DATA_BLOCK DB 1
TITLE =Analog value display
VERSION : 0.1


  STRUCT
   CH_0 : INT ; //Channel 0
   CH_1 : INT ; //Channel 1
   CH_2 : INT ; //Channel 2
   CH_3 : INT ; //Channel 3
   CH_4 : INT ; //Channel 4
   CH_5 : INT ; //Channel 5
   CH_6 : INT ; //Channel 6
   CH_7 : INT ; //Channel 7
  END_STRUCT ;
BEGIN
   CH_0 := 0;
   CH_1 := 0;
   CH_2 := 0;
   CH_3 := 0;
   CH_4 := 0;
   CH_5 := 0;
   CH_6 := 0;
   CH_7 := 0;
END_DATA_BLOCK

DATA_BLOCK DB 2
TITLE =Process values
VERSION : 0.1

  STRUCT
   SE_1 : REAL ;    //Voltage Transducer
   SE_2 : REAL ;    //PT100 (4)
   SE_3 : REAL ;    //PT100 (3)
   SE_4 : REAL ;    //PT100 (2)
  END_STRUCT ;
BEGIN
   SE_1 := 0.000000e+000;
   SE_2 := 0.000000e+000;
   SE_3 := 0.000000e+000;
   SE_4 := 0.000000e+000;
END_DATA_BLOCK

FUNCTION FC 1 : VOID
TITLE =Convert analog value display to process values
VERSION : 0.1


VAR_INPUT
  RawValue : INT ;
  Factor : REAL ;
  Offset : REAL ;
  OverFlow : INT ;
  OverRange : INT ;
  UnderRange : INT ;
  UnderFlow : INT ;
END_VAR
VAR_OUTPUT
  MeasuredValue : REAL ;
  Status : WORD ;
END_VAR
VAR_TEMP
  TInt : INT ;
  TDoubleInt : DINT ;
  TFactor : REAL ;
  TOffset : REAL ;
  TFactor1 : DINT ;
  TFactor2 : REAL ;
END_VAR
BEGIN
NETWORK
TITLE =Conversion

      L     #RawValue;
      ITD   ;
      DTR   ;
      L     #Factor;
      *R    ;
      L     #Offset;
      +R    ;
      T     #MeasuredValue;

NETWORK
TITLE =Analog value display monitoring

      L     W#16#0;
      T     #Status;


      L     #RawValue;
      L     #OverFlow;
      >=I   ;
      SPB   m_of;

      L     #RawValue;
      L     #OverRange;
      >=I   ;
      SPB   m_or;

      L     #RawValue;
      L     #UnderFlow;
      <=I   ;
      SPB   m_uf;

      L     #RawValue;
      L     #UnderRange;
      <=I   ;
      SPB   m_ur;

      SPA   end;

m_of: L     W#16#800;
      T     #Status;
      SPA   end;

m_or: L     W#16#400;
      T     #Status;
      SPA   end;

m_uf: L     W#16#200;
      T     #Status;
      SPA   end;

m_ur: L     W#16#100;
      T     #Status;
      SPA   end;

end:  NOP   0;
END_FUNCTION

ORGANIZATION_BLOCK OB 1
TITLE = "Main Program Sweep (Cycle)"
VERSION : 0.1


VAR_TEMP
  OB1_EV_CLASS : BYTE ; //Bits 0-3 = 1 (Coming event), Bits 4-7 = 1 (Event class 1)
  OB1_SCAN_1 : BYTE ;   //1 (Cold restart scan 1 of OB 1), 3 (Scan 2-n of OB 1)
  OB1_PRIORITY : BYTE ; //Priority of OB Execution
  OB1_OB_NUMBR : BYTE ; //1 (Organization block 1, OB1)
  OB1_RESERVED_1 : BYTE ;   //Reserved for system
  OB1_RESERVED_2 : BYTE ;   //Reserved for system
  OB1_PREV_CYCLE : INT ;    //Cycle time of previous OB1 scan (millisec-onds)
  OB1_MIN_CYCLE : INT ; //Minimum cycle time of OB1 (milliseconds)
  OB1_MAX_CYCLE : INT ; //Maximum cycle time of OB1 (milliseconds)
  OB1_DATE_TIME : DATE_AND_TIME ;   //Date and time OB1 started
END_VAR
BEGIN
NETWORK
TITLE =Transfer of channel values into data block DB1

// Channel 0 -> Data block
      L     PIW  352;
      T     DB1.DBW    0;

// Channel 1 -> Data block
      L     PIW  354;
      T     DB1.DBW    2;

// Channel 2 -> Data block
      L     PIW  356;
      T     DB1.DBW    4;

// Channel 3 -> Data block
      L     PIW  358;
      T     DB1.DBW    6;

// Channel 4 -> Data block
      L     PIW  360;
      T     DB1.DBW    8;

// Channel 5 -> Data block
      L     PIW  362;
      T     DB1.DBW   10;

// Channel 6 -> Data block
      L     PIW  364;
      T     DB1.DBW   12;

// Channel 7 -> Data block
      L     PIW  366;
      T     DB1.DBW   14;



NETWORK
TITLE =Converting analog value display -> Measurement value

// Channel 1 : Voltage transducer 1 to 5V

      CALL FC     1 (
           RawValue                 := DB1.DBW    0,
           Factor                   := 1.447000e-004,
           Offset                   := 1.000000e+000,
           OverFlow                 := 32512,
           OverRange                := 27649,
           UnderRange               := -1,
           UnderFlow                := -4865,
           MeasuredValue            := DB2.DBD    0,
           Status                   := MW    10);

// Channel 2 : PT100

      CALL FC     1 (
           RawValue                 := DB1.DBW    4,
           Factor                   := 1.000000e-001,
           Offset                   := 0.000000e+000,
           OverFlow                 := 10001,
           OverRange                := 8501,
           UnderRange               := -2001,
           UnderFlow                := -2431,
           MeasuredValue            := DB2.DBD    4,
           Status                   := MW    20);

// Channel 3 : PT100

      CALL FC     1 (
           RawValue                 := DB1.DBW    8,
           Factor                   := 1.000000e-001,
           Offset                   := 0.000000e+000,
           OverFlow                 := 10001,
           OverRange                := 8501,
           UnderRange               := -2001,
           UnderFlow                := -2431,
           MeasuredValue            := DB2.DBD    8,
           Status                   := MW    30);

// Channel 4: PT 100

      CALL FC     1 (
           RawValue                 := DB1.DBW   12,
           Factor                   := 1.000000e-001,
           Offset                   := 0.000000e+000,
           OverFlow                 := 10001,
           OverRange                := 8501,
           UnderRange               := -2001,
           UnderFlow                := -2431,
           MeasuredValue            := DB2.DBD   12,
           Status                   := MW    40);

NETWORK
TITLE = Acknowledge hardware interrupt

      U     M    200.0;
      FP    M    200.1;
      SPBN  m001;
      L     0;
      T     MD   100;
      T     MW   104;
      T     MW   106;
      R     M    200.0;
m001: NOP   0;

END_ORGANIZATION_BLOCK


ORGANIZATION_BLOCK OB 40
TITLE = "Hardware Interrupt"
VERSION : 0.1


VAR_TEMP
  OB40_EV_CLASS : BYTE ;    //Bits 0-3 = 1 (Coming event), Bits 4-7 = 1 (Event class 1)
  OB40_STRT_INF : BYTE ;    //16#41 (OB 40 has started)
  OB40_PRIORITY : BYTE ;    //Priority of OB Execution
  OB40_OB_NUMBR : BYTE ;    //40 (Organization block 40, OB40)
  OB40_RESERVED_1 : BYTE ;  //Reserved for system
  OB40_IO_FLAG : BYTE ; //16#54 (input module), 16#55 (output module)
  OB40_MDL_ADDR : WORD ;    //Base address of module initiating interrupt
  OB40_POINT_ADDR : DWORD ; //Interrupt status of the module
  OB40_DATE_TIME : DATE_AND_TIME ;  //Date and time OB40 started
END_VAR
BEGIN
NETWORK
TITLE =

      L     #OB40_IO_FLAG; // OB40_IO_FLAG    : 16#54 = Input module
      T     MB   104; //                 : 16#55 = Output module

      L     #OB40_MDL_ADDR; // OB40_MDL_ADDR   : Start address of the
      T     MW   106; //                   triggering module

      L     #OB40_POINT_ADDR; // OB40_POINT_ADDR : LB8 = Exceeding high
							 // limit value
      T     MD   100; //

      NOP   0; // OB40_POINT_ADDR : LB9 = Under-run of low limit value
      NOP   0; //

END_ORGANIZATION_BLOCK

ORGANIZATION_BLOCK OB 82
TITLE = "I/O Point Fault"
VERSION : 0.1


VAR_TEMP
  OB82_EV_CLASS : BYTE ;    //16#39, Event class 3, Entering event state,
						   // Internal fault event
  OB82_FLT_ID : BYTE ;  //16#XX, Fault identifcation code
  OB82_PRIORITY : BYTE ;    //Priority of OB Execution
  OB82_OB_NUMBR : BYTE ;    //82 (Organization block 82, OB82)
  OB82_RESERVED_1 : BYTE ;  //Reserved for system
  OB82_IO_FLAG : BYTE ; //Input (01010100), Output (01010101)
  OB82_MDL_ADDR : WORD ;    //Base address of module with fault
  OB82_MDL_DEFECT : BOOL ;  //Module defective
  OB82_INT_FAULT : BOOL ;   //Internal fault
  OB82_EXT_FAULT : BOOL ;   //External fault
  OB82_PNT_INFO : BOOL ;    //Point information
  OB82_EXT_VOLTAGE : BOOL ; //External voltage low
  OB82_FLD_CONNCTR : BOOL ; //Field wiring connector missing
  OB82_NO_CONFIG : BOOL ;   //Module has no configuration data
  OB82_CONFIG_ERR : BOOL ;  //Module has configuration error
  OB82_MDL_TYPE : BYTE ;    //Type of module
  OB82_SUB_MDL_ERR : BOOL ; //Sub-Module is missing or has error
  OB82_COMM_FAULT : BOOL ;  //Communication fault
  OB82_MDL_STOP : BOOL ;    //Module is stopped
  OB82_WTCH_DOG_FLT : BOOL ;    //Watch dog timer stopped module
  OB82_INT_PS_FLT : BOOL ;  //Internal power supply fault
  OB82_PRIM_BATT_FLT : BOOL ;   //Primary battery is in fault
  OB82_BCKUP_BATT_FLT : BOOL ;  //Backup battery is in fault
  OB82_RESERVED_2 : BOOL ;  //Reserved for system
  OB82_RACK_FLT : BOOL ;    //Rack fault, only for bus interface module
  OB82_PROC_FLT : BOOL ;    //Processor fault
  OB82_EPROM_FLT : BOOL ;   //EPROM fault
  OB82_RAM_FLT : BOOL ; //RAM fault
  OB82_ADU_FLT : BOOL ; //ADU fault
  OB82_FUSE_FLT : BOOL ;    //Fuse fault
  OB82_HW_INTR_FLT : BOOL ; //Hardware interupt input in fault
  OB82_RESERVED_3 : BOOL ;  //Reserved for system
  OB82_DATE_TIME : DATE_AND_TIME ;  //Date and time OB82 started
END_VAR
BEGIN
END_ORGANIZATION_BLOCK

